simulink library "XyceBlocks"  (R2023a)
settings: Solver=VariableStepAuto  StartTime=0.0  StopTime=10.0  RelTol=1e-3
undefined symbols (not defined in the file or in its folder): ADC1, ADC2, ADCn, multiDac, node, pick_a_circuit, v

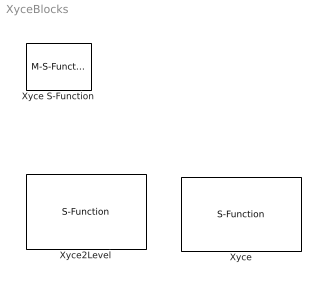
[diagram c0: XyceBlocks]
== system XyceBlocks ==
  Xyce : S-Function  Commented=on  FunctionName=xyce_sfunction  Parameters=UserSelectedXyceInputFileName,InputNames,OutputNames  SFunctionDeploymentMode=off  EnableBusSupport=off  mask{UserSelectedXyceInputFileName=pick_a_circuit.cir, InputNames=DAC1,DAC2,...,DACn, Parameters, OutputNames=ADC1,ADC2,...,ADCn, v(node)}
      mask prompts: UserSelectedXyceInputFileName "Xyce Input Filename"; InputNames "Input DAC Names"; OutputNames "Output ADC Names"
      mask init:
      | % Need to add the location of the simulink interface library to Matlabs search path.
      | %
      | % dumb way to do it for now.
      | %xyce_home = getenv('XYCE_HOME')
      | %xyce_lib_path = [xyce_home filesep 'lib' ]
      | %addpath(xyce_lib_path)
      | 
      | % 
      | % a better way would be it 
      | % 1. check for xyce_sfunction.mexmaci64 where the suffix will be platform dependent 
      | %    as in mexw64 (windows), mexa64 (linux) and mexmaci64 (MacOS)
      | % 2. if the file is not found then use pathtool to let the use select the path.
      | set_param( gcb, 'UserData', ['circiut.cir'] );
  Xyce S-Function : M-S-Function  FunctionName=XyceSFunctionImp  Parameters=XyceInputFileName,WorkingDirectory,NumberOfInputs,NumberOfOutputs,InputNames,OutputNames  mask{XyceInputFileName=multiDac.cir, WorkingDirectory=/Users/rlschie/src/XyceDevelopment/Xyce_Regression/Netlists/SIMULINK/, XyceInputPortNames=, XyceOutputPortNames=, NumberOfInputs=2, NumberOfOutputs=1, InputNames={ '-', 'TEMP'; '1', 'YDAC!DAC_DRIVER1'; '2', 'YDAC!DAC_DRIVER2'; '-', 'YDAC!DAC_DRIVER3' }, OutputNames={ '1', 'YADC!ADC2'; '-', 'TEMP'; '-', 'YADC!ADC1' }}
      mask prompts: XyceInputFileName "Xyce Input Filename"; WorkingDirectory "Working Directory"; XyceInputPortNames "Xyce Input Port Names"; XyceOutputPortNames "Xyce Output Port Names"; NumberOfInputs "Number of Inputs"; NumberOfOutputs "Number of Outputs"; InputNames "Input Names"; OutputNames "Output Names"
  Xyce2Level : S-Function  Commented=on  InitFcn=|  FunctionName=xyce2nLv_sfunction  Parameters='resInnerTran.cir'  SFunctionDeploymentMode=off  EnableBusSupport=off
      | % Need to add the location of the simulink interface library to Matlabs search path.
      | %
      | % dumb way to do it for now.
      | addpath('/Users/rlschie/src/XyceDevelopment/BUILD/NormalCmake/utils/SimulinkInterface')
      | % 
      | % a better way would be it 
      | % 1. check for xyce2nLv_sfunction.mexmaci64 where the suffix will be platform dependent 
      | %    as in mexw64 (windows), mexa64 (linux) and mexmaci64 (MacOS)
      | % 2. if th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
